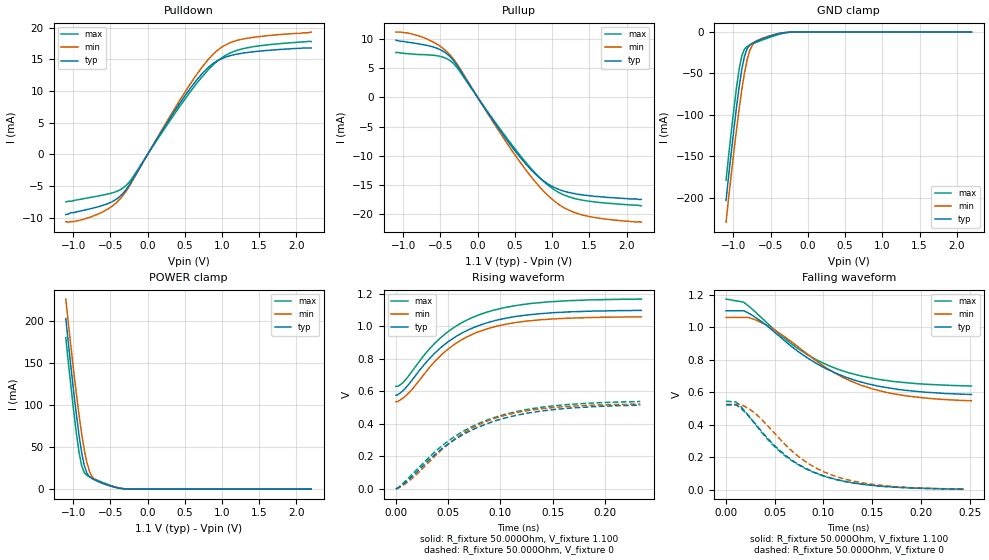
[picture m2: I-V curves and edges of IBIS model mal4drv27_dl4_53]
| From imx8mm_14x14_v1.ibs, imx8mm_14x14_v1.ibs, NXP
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[Model] mal4drv27_dl4_53
Model_type   I/O
Polarity   Non-Inverting
Enable   Active-High
C_comp   1.539pF   1.529pF   1.545pF
C_comp_pullup   679.378fF   664.447fF   683.692fF
C_comp_pulldown 805.519fF   796.861fF   822.151fF
Vinh = 327.000mV
Vinl = 207.000mV
Vmeas = 267.000mV
Vref = 267.000mV
Rref = 50Ohms
Cref = 5pF
[Model Spec]
Vinh   327.000mV   317.000mV   344.000mV
Vinl   207.000mV   197.000mV   224.000mV
Vmeas   267.000mV   257.000mV   284.000mV
Vref   267.000mV   257.000mV   284.000mV
D_overshoot_ampl_h 0.3 NA   NA
D_overshoot_ampl_l 0.3 NA   NA
D_overshoot_area_l 100.000m NA   NA
D_overshoot_area_h 100.000m NA   NA
|[Receiver Thresholds]
|Vth = 267.000mV
|Vth_min = 257.000mV
|Vth_max = 284.000mV
|Vinh_ac = 600.000mV
|Vinh_dc = 600.000mV
|Vinl_ac = -600.000mV
|Vinl_dc = -600.000mV
|Tslew_ac = 5.000ns
|Threshold_sensitivity = 0.5
|Reference_supply Pullup_ref
[Temperature Range]   25.000   125.000   -40.000
[Voltage Range]   1.100V   1.060V   1.170V
[GND Clamp Reference]   0.00V   0.00V   0.00V
|[C Comp Corner]
|| variable   typ   min   max
|C_comp 1.545pF   1.529pF   1.539pF
|C_comp_pullup 683.692fF   664.447fF   679.378fF
|C_comp_pulldown 805.519fF   822.151fF   796.861fF
[Pulldown Reference]   0.00V   0.00V   0.00V
[POWER Clamp Reference]   1.100V   1.060V   1.170V
[Pullup Reference]   1.100V   1.060V   1.170V
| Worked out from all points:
|   slope of the pulldown table from 0 to 0.165 V, typ, clamps not added: 52 ohm
|   slope of the pullup table from 0 to 0.165 V, typ, clamps not added: 52.1 ohm
|   GND clamp passes 1 mA (typ) near -0.34 V on its own axis
|   POWER clamp passes 1 mA (typ) near -0.37 V on its own axis
|   rising waveform, R_fixture 50.000Ohm, V_fixture 1.100: 20-80 % time 58ps typ, 55ps min, 58.4ps max; typ from 0.576 V to 1.1 V
|   rising waveform, R_fixture 50.000Ohm, V_fixture 0: 20-80 % time 72.2ps typ, 65.2ps min, 72ps max; typ from -0.002 V to 0.514 V
|   falling waveform, R_fixture 50.000Ohm, V_fixture 1.100: 20-80 % time 80.4ps typ, 79.3ps min, 78.1ps max; typ from 1.1 V to 0.585 V
|   falling waveform, R_fixture 50.000Ohm, V_fixture 0: 20-80 % time 62.3ps typ, 62.6ps min, 62.2ps max; typ from 0.522 V to 0.003 V
[GND Clamp]
-1.099V   -203.4mA   -229.8mA   -179.1mA
-1.028V   -144.6mA   -171.6mA   -119.9mA
-957.3mV  -89.96mA   -117.2mA   -66.34mA
-921.8mV  -65.62mA   -92.07mA   -44.23mA
-886.4mV  -44.77mA   -69.12mA   -28.39mA
-850.9mV  -29.17mA   -49.17mA   -20.45mA
-815.5mV  -19.93mA   -33.26mA   -17.37mA
-780mV    -15.54mA   -22.17mA   -15.71mA
-709.1mV  -11.77mA   -11.95mA   -13.05mA
-460.9mV  -3.594mA   -3.176mA   -4.769mA
-212.7mV  -39.63uA   -70.42uA   -94.27uA
2.198V    74.25nA    840.4nA    20.58nA
[Power Clamp]
-1.098V   203.2mA    226.4mA    180.4mA
-1.027V   144mA      168.2mA    120.9mA
-956.4mV  89.16mA    113.9mA    66.8mA
-920.9mV  64.74mA    88.96mA    44.41mA
-885.5mV  43.86mA    66.33mA    28.14mA
-850mV    28.29mA    46.87mA    19.77mA
-814.5mV  19.12mA    31.59mA    16.46mA
-779.1mV  14.74mA    21.12mA    14.69mA
-708.2mV  10.9mA     11.5mA     11.88mA
-530.9mV  4.726mA    4.702mA    5.575mA
-282.7mV  125.9uA    313.7uA    153.4uA
2.199V    -42.87nA   -857.3nA   -9.404nA
[Pulldown]
-1.099V   -9.5mA     -10.6mA    -7.5mA
-921.8mV  -8.99mA    -10.43mA   -7.13mA
-602.7mV  -8.047mA   -9.068mA   -6.426mA
-425.5mV  -7.113mA   -7.678mA   -5.883mA
-283.6mV  -5.465mA   -5.723mA   -4.843mA
212.7mV   4.069mA    4.29mA     3.799mA
531.8mV   9.746mA    10.38mA    9.21mA
744.5mV   12.9mA     13.96mA    12.42mA
957.3mV   14.9mA     16.6mA     14.91mA
1.099V    15.55mA    17.57mA    15.95mA
1.312V    16.04mA    18.27mA    16.76mA
2.198V    16.8mA     19.3mA     17.8mA
[Pullup]
-1.098V   9.8mA      11.2mA     7.7mA
-672.7mV  8.896mA    9.968mA    7.289mA
-495.5mV  8.144mA    8.697mA    7.013mA
-353.6mV  6.755mA    7.022mA    6.138mA
-247.3mV  4.915mA    5.159mA    4.588mA
213.6mV   -4.077mA   -4.35mA    -3.868mA
532.7mV   -9.662mA   -10.43mA   -9.333mA
816.4mV   -13.62mA   -15.11mA   -13.54mA
1.029V    -15.45mA   -17.77mA   -15.84mA
1.206V    -16.25mA   -19.23mA   -16.96mA
1.419V    -16.74mA   -20.2mA    -17.65mA
2.199V    -17.5mA    -21.4mA    -18.6mA
[Ramp]
R_load=50.000Ohm
dV/dt_r   313.140mV/67.500ps  314.248mV/61.500ps  324.240mV/67.500ps
dV/dt_f   313.140mV/74.500ps  314.248mV/74.500ps  324.240mV/72.500ps
[Rising waveform]
R_fixture=50.000Ohm
V_fixture=1.100
V_fixture_min=1.060
V_fixture_max=1.170
0s        576mV      535.7mV    630.5mV
5ps       594.1mV    550.1mV    644.2mV
12ps      640.3mV    587.3mV    692.9mV
30ps      786mV      729.8mV    845.5mV
45ps      880mV      832.9mV    941.8mV
62ps      954.3mV    914.1mV    1.018V
83ps      1.013V     975.5mV    1.079V
111ps     1.057V     1.02V      1.124V
144ps     1.081V     1.043V     1.15V
235ps     1.098V     1.058V     1.168V
[Rising waveform]
R_fixture=50.000Ohm
V_fixture=0
0s        -1.881mV   -2.266mV   -3.003mV
16ps      78.11mV    66mV       92.04mV
35ps      196.7mV    185mV      213.5mV
49ps      270.3mV    269.5mV    288.6mV
70ps      352.4mV    363.8mV    373.2mV
93ps      413.3mV    429.6mV    435.9mV
117ps     454.3mV    470.4mV    477.1mV
148ps     485.3mV    498.4mV    508mV
181ps     502.7mV    512.4mV    525.6mV
234ps     514.4mV    520.9mV    536.9mV
[Falling waveform]
R_fixture=50.000Ohm
V_fixture=1.100
V_fixture_min=1.060
V_fixture_max=1.170
0s        1.101V     1.06V      1.173V
18ps      1.101V     1.06V      1.154V
24ps      1.083V     1.059V     1.126V
41ps      1.014V     1.014V     1.032V
61ps      911.7mV    937.6mV    926mV
80ps      824.8mV    850.2mV    843.7mV
113ps     715.7mV    713.2mV    744.9mV
137ps     664.9mV    645.9mV    701.5mV
171ps     621.5mV    590.6mV    666.4mV
252ps     585.4mV    546.9mV    637.7mV
[Falling waveform]
R_fixture=50.000Ohm
V_fixture=0
0s        521.7mV    524.5mV    543.8mV
10ps      521.7mV    524.5mV    539.5mV
24ps      447.6mV    495.9mV    448.4mV
42ps      320.2mV    397.2mV    313.9mV
59ps      220.8mV    287.5mV    215.5mV
74ps      156.5mV    205.6mV    153.3mV
93ps      100.5mV    130.7mV    98.28mV
117ps     57.04mV    72.69mV    56.07mV
149ps     26.68mV    33.2mV     26.36mV
244ps     2.724mV    3.363mV    2.825mV
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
